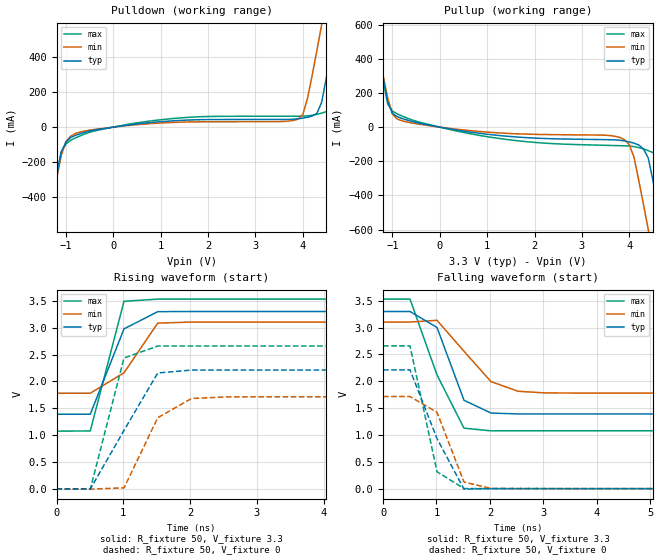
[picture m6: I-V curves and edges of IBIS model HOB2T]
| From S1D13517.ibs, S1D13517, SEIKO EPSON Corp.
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[Model]   HOB2T
Model_type Output
Polarity Non-Inverting
C_comp   5p   4p   6p
[Temperature Range] 50   100   0
[Voltage Range]   3.3   3.0   3.6
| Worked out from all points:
|   slope of the pulldown table from 0 to 0.495 V, typ, clamps not added: 27.1 ohm
|   slope of the pullup table from 0 to 0.495 V, typ, clamps not added: 21.5 ohm
|   falling waveform, R_fixture 50, V_fixture 3.3: 20-80 % time 427ps typ, 704ps min, 610ps max; typ from 3.3 V to 1.39 V
|   falling waveform, R_fixture 50, V_fixture 0: 20-80 % time 593ps typ, 400ps min, 344ps max; typ from 2.21 V to 0 V
|   rising waveform, R_fixture 50, V_fixture 3.3: 20-80 % time 365ps typ, 525ps min, 309ps max; typ from 1.39 V to 3.3 V
|   rising waveform, R_fixture 50, V_fixture 0: 20-80 % time 622ps typ, 446ps min, 331ps max; typ from 0 V to 2.21 V
[Pullup]
-3.3V     3.709A     3.41A      4.072A
-1.4V     610.1mA    596.5mA    627.8mA
-1.1V     146.2mA    169.6mA    135.3mA
-1V       80.25mA    75.92mA    93.36mA
-800mV    50.98mA    37.1mA     65.38mA
1.3V      -50.18mA   -34.56mA   -68.1mA
3.9V      -80.77mA   -73.51mA   -109.4mA
4.1V      -93.88mA   -176mA     -113.8mA
4.4V      -180mA     -598.3mA   -137.7mA
4.7V      -628.2mA   -1.038A    -208mA
5V        -1.114A    -1.478A    -671.6mA
6.6V      -3.721A    -3.84A     -3.587A
[Pulldown]
-3.3V     -3.695A    -3.386A    -4.091A
-1.4V     -600.2mA   -585.7mA   -625.9mA
-1.1V     -142.7mA   -160.1mA   -140.8mA
-1V       -84.36mA   -82.41mA   -95.53mA
-800mV    -46.78mA   -36.14mA   -61.66mA
1.2V      35.16mA    26.31mA    47.77mA
3.9V      47.68mA    45.88mA    62.66mA
4.1V      56.63mA    165.1mA    64.29mA
4.4V      143.7mA    588.9mA    80.26mA
4.7V      604.9mA    1.03A      140mA
5V        1.092A     1.472A     628.5mA
6.6V      3.698A     3.837A     3.528A
[Falling Waveform]
R_fixture=50
V_fixture=3.3
0s        3.3V       3.103V     3.531V
505.1ps   3.3V       3.103V     3.532V
1.01ns    3.003V     3.136V     2.119V
1.515ns   1.647V     2.559V     1.126V
2.02ns    1.408V     1.994V     1.077V
2.525ns   1.392V     1.814V     1.077V
3.03ns    1.391V     1.783V     1.077V
3.535ns   1.391V     1.781V     1.077V
50ns      1.391V     1.781V     1.077V
[Falling Waveform]
R_fixture=50
V_fixture=0
0s        2.212V     1.715V     2.659V
505.1ps   2.212V     1.716V     2.659V
1.01ns    933.7mV    1.422V     315.6mV
1.515ns   -10.01mV   122.9mV    1.365mV
2.02ns    458.8uV    4.018mV    5.277uV
2.525ns   4.669uV    705.8uV    11.69uV
50ns      10.18uV    -948.7nV   -2.455uV
[Rising Waveform]
R_fixture=50
V_fixture=3.3
0s        1.391V     1.781V     1.077V
505.1ps   1.392V     1.781V     1.081V
1.01ns    2.978V     2.162V     3.49V
1.515ns   3.297V     3.085V     3.53V
2.02ns    3.3V       3.104V     3.531V
50ns      3.3V       3.103V     3.531V
[Rising Waveform]
R_fixture=50
V_fixture=0
0s        0V         0V         0V
505.1ps   8.426uV    -7.448uV   -1.15mV
1.01ns    1.092V     23.03mV    2.436V
1.515ns   2.157V     1.327V     2.659V
2.02ns    2.212V     1.683V     2.659V
2.525ns   2.212V     1.712V     2.659V
50ns      2.212V     1.715V     2.659V
[Ramp]
R_load=50
dV/dt_r   1.327E+0/2.893E-10   1.029E+0/3.836E-10   1.595E+0/2.053E-10
dV/dt_f   1.145E+0/4.208E-10   8.802E-1/5.351E-10   1.437E+0/3.294E-10
|[End   HOB2T
